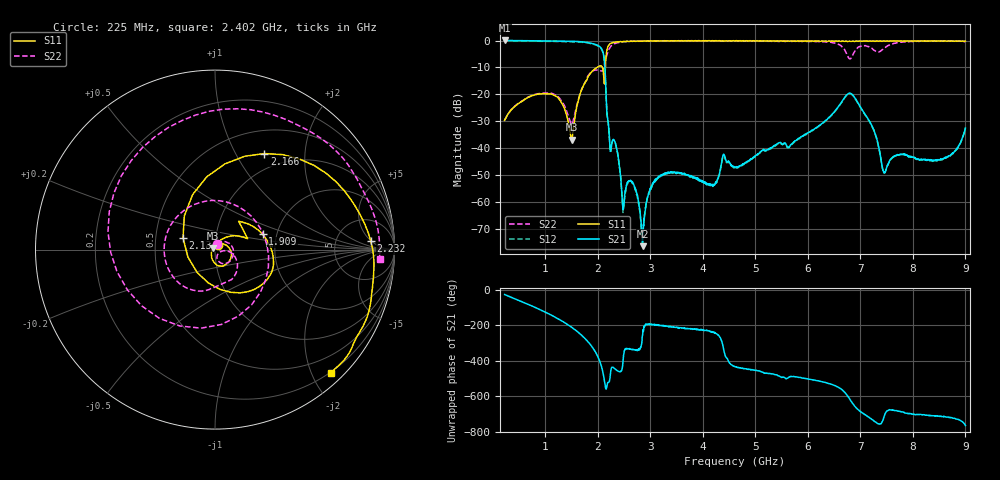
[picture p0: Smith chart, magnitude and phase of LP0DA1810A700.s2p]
!Agilent Technologies,E8358A,US41080443,A.07.50.56
!Agilent E8358A: A.07.50.56
!Date: Wednesday, August 24, 2016 14:41:40
!Correction: S11(Full 2 Port(1,2))
!S21(Full 2 Port(1,2))
!S12(Full 2 Port(1,2))
!S22(Full 2 Port(1,2))
!S2P File: Measurements: S11, S21, S12, S22:
# Hz S  dB  R 50
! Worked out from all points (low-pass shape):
!   1601 points, 225 MHz to 9 GHz, reference 50 ohm
!   highest |S21| = 0.03 dB at 230.5 MHz (marker M1); lowest = -76.4 dB at 2.852 GHz (marker M2)
!   |S21| within 3 dB of the highest: start of sweep to 2.067 GHz
!   lowest |S11| = -36.8 dB at 1.503 GHz (marker M3), VSWR 1.03, Z = 48.8 + j0.711 ohm
!   |S11| at or under -10 dB: start of sweep to 1.984 GHz; 2.087 GHz to 2.144 GHz (56.67 MHz wide, 2.68 % of centre)
!   |S22| runs from -31.0 to 0.0 dB; largest |S21 - S12| = 0.019
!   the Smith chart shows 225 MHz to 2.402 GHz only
!   S11 on the Smith chart (normalised r, x): 225 MHz: 1.03, +0.06; 1.909 GHz: 1.69, +0.31; 2.134 GHz: 0.69, +0.09; 2.166 GHz: 0.79, +1.32; 2.232 GHz: 12, +5; 2.402 GHz: 0.18, -2.31
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2.25e8  -29.63 57.6  0.03 -27.0  -0.12 -26.8  -29.56 68.9
2.304844e8  -29.42 56.7  0.03 -27.6  -0.13 -27.4  -29.36 68.0
8.776406e8  -19.90 -32.0  -0.11 -108.9  -0.27 -108.7  -19.72 -5.5
1.502859e9  -36.80 149.7  -0.26 148.5  -0.41 148.7  -30.94 -45.3
1.689328e9  -18.39 39.6  -0.48 104.3  -0.62 104.5  -18.29 -21.2
1.908703e9  -11.09 17.8  -1.17 30.8  -1.34 31.0  -11.24 -137.4
2.133562e9  -14.42 159.7  -9.66 -168.7  -9.82 -168.4  -8.66 -56.4
2.166469e9  -4.41 62.8  -24.44 166.5  -24.58 166.6  -5.76 -142.6
2.232281e9  -1.22 3.2  -40.10 -135.8  -40.23 -136.3  -2.59 104.4
2.402297e9  -0.49 -46.6  -45.12 -101.0  -45.32 -100.8  -0.73 -3.4
2.852016e9  -0.26 -94.3  -76.42 101.3  -71.45 109.1  -0.22 -81.4
3.153656e9  -0.16 -110.7  -50.51 161.1  -50.84 160.9  -0.11 -104.9
4.6125e9  -0.15 -145.0  -47.03 -72.6  -47.49 -71.8  -0.14 -178.9
6.076828e9  -0.13 -178.4  -33.30 -146.8  -33.66 -147.1  -0.39 75.8
6.603328e9  -0.19 166.6  -23.93 166.2  -24.14 167.0  -1.66 4.6
6.745922e9  -0.31 162.6  -20.11 125.9  -20.21 126.5  -5.24 -71.8
6.855609e9  -0.19 160.4  -20.19 77.8  -20.38 78.1  -5.30 157.3
6.992719e9  -0.17 156.6  -24.39 35.5  -24.62 35.9  -2.23 76.5
7.184672e9  -0.15 152.1  -30.34 -3.0  -30.55 -2.4  -2.62 4.3
7.343719e9  -0.25 148.7  -39.03 -36.0  -39.15 -35.8  -4.24 -98.9
7.541156e9  -0.26 144.2  -45.41 41.1  -45.44 42.7  -1.79 153.9
9e9  -0.20 118.0  -32.53 -44.6  -32.70 -44.8  -0.55 45.4
